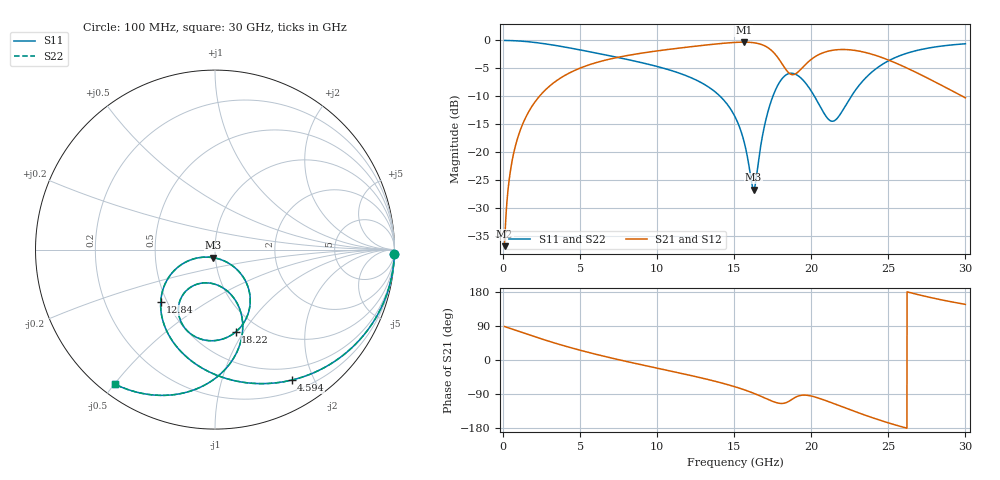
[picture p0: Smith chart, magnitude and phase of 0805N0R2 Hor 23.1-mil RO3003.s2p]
# GHz S MA R 50
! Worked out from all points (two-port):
!   3201 points, 100 MHz to 30 GHz, reference 50 ohm
!   highest |S21| = -0.30 dB at 15.62 GHz (marker M1); lowest = -36.9 dB at 100 MHz (marker M2)
!   |S21| within 3 dB of the highest: 6.98 GHz to 17.89 GHz (10.91 GHz wide, 87.7 % of centre); 20.04 GHz to 24.82 GHz (4.778 GHz wide, 21.3 % of centre)
!   lowest |S11| = -26.7 dB at 16.26 GHz (marker M3), VSWR 1.10, Z = 49 - j4.44 ohm
!   |S11| at or under -10 dB: 14.08 GHz to 17.51 GHz (3.426 GHz wide, 21.7 % of centre); 20.2 GHz to 22.6 GHz (2.391 GHz wide, 11.2 % of centre)
!   |S22| runs from -26.7 to 0.0 dB; largest |S21 - S12| = 0
!   S11 on the Smith chart (normalised r, x): 100 MHz: 1, -81; 4.594 GHz: 0.34, -1.70; 12.84 GHz: 0.46, -0.33; 18.22 GHz: 0.78, -0.92; 30 GHz: 0.04, -0.50
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0.1  0.9998 -1.4  0.01435 88.2  0.01435 88.2  0.9998 -1.4
0.3335938  0.9987 -4.7  0.0476 85.1  0.0476 85.1  0.9987 -4.7
0.5391563  0.9969 -7.6  0.07673 82.2  0.07673 82.2  0.9969 -7.6
1.296  0.9831 -18.2  0.1814 71.7  0.1814 71.7  0.9831 -18.2
2.613469  0.9377 -35.8  0.3455 54.1  0.3455 54.1  0.9377 -35.8
4.594344  0.8432 -59.6  0.5347 30.2  0.5347 30.2  0.8432 -59.6
5.089563  0.8183 -65.0  0.5716 24.8  0.5716 24.8  0.8183 -65.0
7.537625  0.6998 -89.2  0.7101 0.5  0.7101 0.5  0.6998 -89.2
10.06978  0.5809 -111.7  0.8086 -22.2  0.8086 -22.2  0.5809 -111.7
12.84488  0.4198 -136.1  0.8998 -47.1  0.8998 -47.1  0.4198 -136.1
15.05  0.2073 -155.8  0.9604 -70.7  0.9604 -70.7  0.2073 -155.8
15.61997  0.1267 -156.3  0.9657 -78.2  0.9657 -78.2  0.1267 -156.3
16.25534  0.04601 -100.6  0.9546 -87.7  0.9546 -87.7  0.04601 -100.6
17.19906  0.2331 -45.1  0.8593 -104.1  0.8593 -104.1  0.2331 -45.1
18.21753  0.4731 -75.9  0.5842 -114.2  0.5842 -114.2  0.4731 -75.9
19.21731  0.4747 -109.7  0.5337 -94.3  0.5337 -94.3  0.4747 -109.7
20.03956  0.3448 -124.5  0.6838 -95.4  0.6838 -95.4  0.3448 -124.5
21.46916  0.1901 -93.6  0.8201 -115.1  0.8201 -115.1  0.1901 -93.6
23.23513  0.4168 -68.6  0.7959 -141.9  0.7959 -141.9  0.4168 -68.6
25.01978  0.6581 -84.1  0.6667 -166.1  0.6667 -166.1  0.6581 -84.1
27.23425  0.8359 -105.1  0.4831 169.6  0.4831 169.6  0.8359 -105.1
30  0.9339 -126.4  0.3061 146.8  0.3061 146.8  0.9339 -126.4
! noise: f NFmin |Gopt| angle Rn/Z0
0.1  0.01532  0.9959  0.635  0.8535
3.417  0.009893  0.8101  23.18  0.01042
6.743  0.01424  0.7488  42.26  0.009963
10.06  0.01833  0.7206  59.9  0.009841
13.39  0.02518  0.7353  75.72  0.01201
16.7  0.07806  0.888  90.29  0.07565
20.03  0.2036  0.9486  105.1  0.3293
23.35  0.126  0.9077  118.7  0.07849
26.67  0.129  0.8998  131.3  0.04847
30  0.1533  0.9073  143.4  0.03659
